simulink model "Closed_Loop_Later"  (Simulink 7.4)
settings: Solver=ode45  StartTime=0.0  StopTime=10.0  RelTol=1e-3
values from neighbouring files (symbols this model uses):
  Al = Au([1,2,5,6,8],[1,2,5,6,8])    [Split.m]
  Bl = Bu([1,2,5,6,8],                  [5,6,7,8,   9,11,14,19,20,21,22,24,26,28,29,30,35,36,37,38,39,40,41,42,43])    [Split.m]
  Cl = Cu([1,2,5,6,8,11,13,   15,17,20,25,26,27,28,30,32,34,35,36,41,42,43,44,45,46,47,48,49],         [1,2,5,6,8])    [Split.m]
  Dl = Du([1,2,5,6,8,11,13,   15,17,20,25,26,27,28,30,32,34,35,36,41,42,43,44,45,46,47,48,49],                  [5,6,7,8,   9,11,14,19,20,21,22,24,26,28,29,30,35,36,37,38,39,40,41,42,43])    [Split.m]
  nlu = 21    [run.m]
undefined symbols (not defined in the file or in its folder): Kl

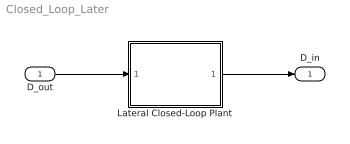
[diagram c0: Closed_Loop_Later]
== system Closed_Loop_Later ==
  D_out : Inport  OutDataType=sfix(16)  OutScaling=2^0
  Lateral Closed-Loop Plant : Subsystem
  D_in : Outport  OutDataType=sfix(16)  OutScaling=2^0
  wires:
  Lateral Closed-Loop Plant/1(D_in) -> D_in/1
  D_out/1 -> Lateral Closed-Loop Plant/1(D_out)

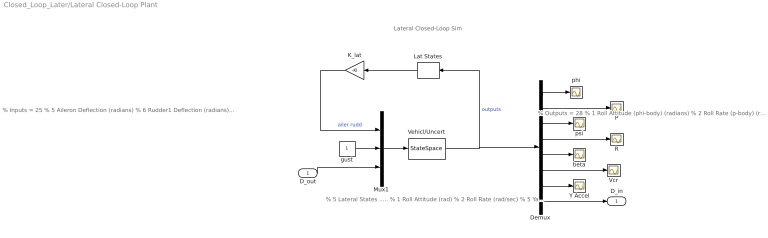
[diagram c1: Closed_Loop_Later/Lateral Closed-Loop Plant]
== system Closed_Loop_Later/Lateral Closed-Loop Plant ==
  note: Lateral Closed-Loop Sim
  note: % 5 Lateral States ..... % 1 Roll Attitude (rad) % 2 Roll Rate (rad/sec) % 5 Yaw Attitude (rad) % 6 Yaw Rate (rad/sec) % 8 Beta (rad)
  note: % Inputs = 25 % 5 Aileron Deflection (radians) % 6 Rudder1 Deflection (radians) % 7 Rudder2 Deflection (radians) % 8 Wind Gust Azim, Elev Angles=(-135.0 90.0) (deg) % Lateral Variations= 21 % 9 Cl_beta : -20.000 % Variation % 11 Cn_beta : 30.303 % Variation % 14 Cy_beta : -14.286 % Variation % 19 Cn_p : 54.348 % Variation % 20 Cn_r : -20.408 % Variation % 21 Cl_p : -33.333 % Variation % 22 Cl_r : 25.000 % Variation % 24 I_xx : 2.857 % Variation % 26 I_zz : 3.030 % Variation % 28 Xcg locat: -1.766 % Variation % 29 Ycg locat: 0.5000 Addit. Variat. % 30 Zcg locat: 0.5000 Addit. Variat. % 35 Cy_surf 2: 500.000 % Variation % 36 Cl_surf 2: 15.000 % Variation % 37 Cn_surf 2: -650.000 % Variation % 38 Cy_surf 3: 10.750 % Variation % 39 Cl_surf 3: 40.000 % Variation % 40 Cn_surf 3: -10.000 % Variation % 41 Cy_surf 4: 5.000 % Variation % 42 Cl_surf 4: 6.250 % Variation % 43 Cn_surf 4: 6.000 % Variation
  note: % Outputs = 28 % 1 Roll Attitude (phi-body) (radians) % 2 Roll Rate (p-body) (rad/sec) % 5 Yaw Attitude (psi-body) (radians) % 6 Yaw Rate (r-body) (rad/sec) % 8 Angle of sideslip, beta, (radian) % 11 Cross Range Velocity (Vcr) (ft/sec) % 13 CG Acceleration along Y axis, (ft/sec^2) % Lateral Variations= 21 % 15 Cl_beta : -20.000 % Variation % 17 Cn_beta : 30.303 % Variation % 20 Cy_beta : -14.286 % Variation % 25 Cn_p : 54.348 % Variation % 26 Cn_r : -20.408 % Variation % 27 Cl_p : -33.333 % Variation % 28 Cl_r : 25.000 % Variation % 30 I_xx : 2.857 % Variation % 32 I_zz : 3.030 % Variation % 34 Xcg locat: -1.766 % Variation % 35 Ycg locat: 0.5000 Addit. Variat. % 36 Zcg locat: 0.5000 Addit. Variat. % 41 Cy_surf 2: 500.000 % Variation % 42 Cl_surf 2: 15.000 % Variation % 43 Cn_surf 2: -650.000 % Variation % 44 Cy_surf 3: 10.750 % Variation % 45 Cl_surf 3: 40.000 % Variation % 46 Cn_surf 3: -10.000 % Variation % 47 Cy_surf 4: 5.000 % Variation % 48 Cl_surf 4: 6.250 % Variation % 49 Cn_surf 4: 6.000 % Variation
  D_out : Inport  OutDataType=sfix(16)  OutScaling=2^0
  Demux : Demux  Outputs="[1, 1, 1, 1, 1, 1, 1,   nlu]"
  K_lat : Gain  Gain=-Kl  Multiplication=Matrix(K*u)  ParameterDataType=sfix(16)  ParameterScaling=2^0  OutDataType=sfix(16)  OutScaling=2^0
  Lat States : Selector  InputPortWidth=7+nlu  IndexOptions=Index vector (dialog)  Indices=[1,2,3,4,5]  OutputSizes=1
  Mux1 : Mux  Inputs=[3, 1, nlu]
  P : Scope
  R : Scope
  Vcr : Scope
  Vehicl/Uncert : StateSpace  A=Al  B=Bl  C=Cl  D=Dl
  Y Accel : Scope
  beta : Scope
  gust : Constant  OutDataType=sfix(16)  OutScaling=2^0
  phi : Scope
  psi : Scope
  D_in : Outport  OutDataType=sfix(16)  OutScaling=2^0
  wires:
  Vehicl/Uncert/1 -> Demux/1, Lat States/1  "outputs"
  Demux/1 -> phi/1
  Demux/3 -> psi/1
  Demux/4 -> R/1
  Demux/2 -> P/1
  Lat States/1 -> K_lat/1
  D_out/1 -> Mux1/3
  K_lat/1 -> Mux1/1  "ailer rudd"
  Demux/7 -> Y Accel/1
  Demux/8 -> D_in/1
  Demux/5 -> beta/1
  Demux/6 -> Vcr/1
  Mux1/1 -> Vehicl/Uncert/1
  gust/1 -> Mux1/2
